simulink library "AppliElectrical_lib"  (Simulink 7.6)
settings: Solver=ode45  StartTime=0.0  StopTime=10.0  RelTol=1e-3
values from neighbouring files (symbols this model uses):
  A = [1+j -(1-j);1 -2/(1-j)]    [systeme_AX_B_phaseurs.m]
undefined symbols (not defined in the file or in its folder): AppliElectrical, erreur, F, gcbh, Giacolleto_NPN, model_FET_canal_N, nesl_callback, Ohm, PID_analogique, s, Transistor_NPN, V, vb2c, vb2e

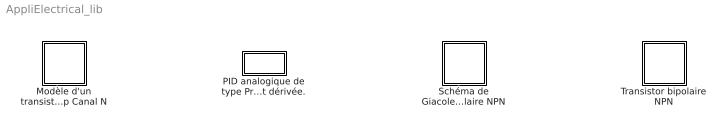
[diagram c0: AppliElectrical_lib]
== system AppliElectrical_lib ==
  Modèle d'un transistor à effet de champ Canal N : Subsystem  DialogController=NetworkEngine.DynNeDlgSource  LoadFcn=nesl_callback('LoadFcn',gcbh);  mask(Modèle d'un
transistor à effet
de champ Canal N){ComponentPath=AppliElectrical.model_FET_canal_N, ClassName=model_FET_canal_N, SchemaVersion=1, g=0.003, g_unit=A/V, rho=1e+6, rho_unit=Ohm, ie_Log=off, vgs_Log=off, is_Log=off, vds_Log=off, LocalVarNames=\, LocalVarDescs=ie\, LocalVarLogging=vgs\}
      mask help: Le modèle qui définit ce transistor spécifie: - la résistance Rgs entre la grille et la source, - la conductance g ou pente g=dId/dVgs, - sa résistance rho en parallèle à la source de courant g Vds.
      mask init:
      | nesl_preinitmask (gcb);
  "PID analogique de type Proportionnel, Intégral et dérivée." : Subsystem  DialogController=NetworkEngine.DynNeDlgSource  LoadFcn=nesl_callback('LoadFcn',gcbh);  mask(PID analogique de
type Proportionnel,
Intégral et dérivée.){ComponentPath=AppliElectrical.PID_analogique, ClassName=PID_analogique, SchemaVersion=1, Kp=10, Kp_unit=1, Ki=0.5, Ki_unit=1/s, Kd=0.01, Kd_unit=s, deriv_Log=off, erreur_Log=off, LocalVarNames=\, LocalVarDescs=deriv\, LocalVarLogging=erreur}
      mask prompts: Kp "Gain proportionnel"; Ki "Gain intégral"; Kd "Gain dérivée"
      mask help: L'entrée, err, de ce composant est l'erreur consigne-sortie. La sortie, cde, est la variation de commande. De fait, ce composant doit être suivi d'un intégrateur pour obtenir la commande à appliquer au processus
      mask init:
      | nesl_preinitmask (gcb);
  Schéma de Giacoletto d'un transistor bipolaire NPN : Subsystem  DialogController=NetworkEngine.DynNeDlgSource  LoadFcn=nesl_callback('LoadFcn',gcbh);  mask(Schéma de Giacoletto
d'un transistor
bipolaire NPN){ComponentPath=AppliElectrical.Giacolleto_NPN, ClassName=Giacolleto_NPN, SchemaVersion=1, Cbe=8e-11, Cbe_unit=F, Cbc=1e-11, Cbc_unit=F, h11=1000, h11_unit=Ohm, rbb=100, rbb_unit=Ohm, h21=100, h21_unit=1, g=1e-5, g_unit=1/Ohm, vb2e_Log=off, vb2c_Log=off, Ib_Log=off, Vbe_Log=off, Ic_Log=off, Vce_Log=off, LocalVarNames=\, LocalVarDescs=vb2e\, LocalVarLogging=vb2c\}
      mask prompts: Cbe "Capacitance Cb'e"; Cbc "Capacitance Cb'c"; h11 "résistance h11"; rbb "résistance rbb'"; h21 "gain en tension Ic=h21 Ib"; g "conductance 1/h22"
      mask help: Le schéma de Giacoletto modélise les transistors en hautes fréquences. Le modèle a besoin des paramètres suivants:
      mask init:
      | nesl_preinitmask (gcb);
  Transistor bipolaire NPN : Subsystem  DialogController=NetworkEngine.DynNeDlgSource  LoadFcn=nesl_callback('LoadFcn',gcbh);  mask(Transistor bipolaire
NPN){ComponentPath=AppliElectrical.Transistor_NPN, ClassName=Transistor_NPN, SchemaVersion=1, s=1e-6, s_unit=1/Ohm, h21=200, h21_unit=1, h12=1e-4, h12_unit=1, h11=1000, h11_unit=Ohm, Ib_Log=off, Vbe_Log=off, Ic_Log=off, Vce_Log=off, LocalVarNames=\, LocalVarDescs=Ib\, LocalVarLogging=Vbe\}
      mask prompts: s "1/h22"; h21 "Gain en courant h21"; h12 "Gain en tension inverse"; h11 "Résistance d'entrée h11"
      mask help: Le modèle qui définit ce transistor spécifie: - la résistance 1/h22 (s) entre le collecteur et l'émetteur - le gain en courant h21, - le paramètre h12, amplification inverse en tension - sa résistance d'entrée h11.
      mask init:
      | nesl_preinitmask (gcb);

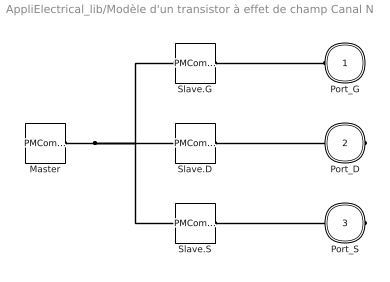
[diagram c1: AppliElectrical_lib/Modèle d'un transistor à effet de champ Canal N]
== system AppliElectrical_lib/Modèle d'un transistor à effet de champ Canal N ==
  Master : PMComponent  Tag=AppliElectrical.model_FET_canal_N  PhysicalDomain=network_engine_domain  SubClassName=master  LeftPortType=generic  RightPortType=generic  RConnTagsString=RConn1
  Slave.D : PMComponent  Tag=D  PhysicalDomain=network_engine_domain  SubClassName=terminal  LeftPortType=generic  RightPortType=foundation.electrical.electrical  LConnTagsString=LConn1  RConnTagsString=RConn1
  Slave.G : PMComponent  Tag=G  PhysicalDomain=network_engine_domain  SubClassName=terminal  LeftPortType=generic  RightPortType=foundation.electrical.electrical  LConnTagsString=LConn1  RConnTagsString=RConn1
  Slave.S : PMComponent  Tag=S  PhysicalDomain=network_engine_domain  SubClassName=terminal  LeftPortType=generic  RightPortType=foundation.electrical.electrical  LConnTagsString=LConn1  RConnTagsString=RConn1
  Port_G : PMIOPort  Tag=G  Port=1  Side=Left
  Port_D : PMIOPort  Tag=D  Port=2  Side=Right
  Port_S : PMIOPort  Tag=S  Port=3  Side=Right
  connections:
  Slave.G/RConn1 -- Port_G/RConn1
  Slave.G/LConn1 -- Slave.D/LConn1 -- Master/RConn1 -- Slave.S/LConn1
  Slave.D/RConn1 -- Port_D/RConn1
  Slave.S/RConn1 -- Port_S/RConn1

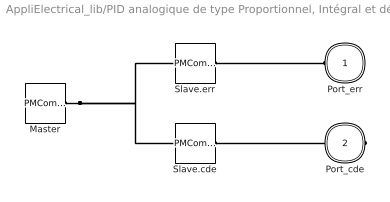
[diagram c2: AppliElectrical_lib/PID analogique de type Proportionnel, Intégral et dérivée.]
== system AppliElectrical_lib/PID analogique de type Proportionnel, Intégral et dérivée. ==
  Master : PMComponent  Tag=AppliElectrical.PID_analogique  PhysicalDomain=network_engine_domain  SubClassName=master  LeftPortType=generic  RightPortType=generic  RConnTagsString=RConn1
  Slave.cde : PMComponent  Tag=cde  PhysicalDomain=network_engine_domain  SubClassName=output  LeftPortType=generic  RightPortType=output  LConnTagsString=LConn1  RConnTagsString=RConn1
  Slave.err : PMComponent  Tag=err  PhysicalDomain=network_engine_domain  SubClassName=input  LeftPortType=generic  RightPortType=input  LConnTagsString=LConn1  RConnTagsString=RConn1
  Port_err : PMIOPort  Tag=err  Port=1  Side=Left
  Port_cde : PMIOPort  Tag=cde  Port=2  Side=Right
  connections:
  Slave.err/RConn1 -- Port_err/RConn1
  Master/RConn1 -- Slave.err/LConn1 -- Slave.cde/LConn1
  Slave.cde/RConn1 -- Port_cde/RConn1

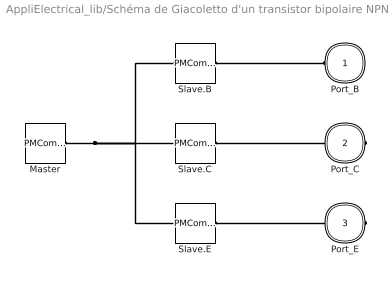
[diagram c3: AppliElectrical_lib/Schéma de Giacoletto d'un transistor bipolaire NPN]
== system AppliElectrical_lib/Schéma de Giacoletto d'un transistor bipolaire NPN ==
  Master : PMComponent  Tag=AppliElectrical.Giacolleto_NPN  PhysicalDomain=network_engine_domain  SubClassName=master  LeftPortType=generic  RightPortType=generic  RConnTagsString=RConn1
  Slave.B : PMComponent  Tag=B  PhysicalDomain=network_engine_domain  SubClassName=terminal  LeftPortType=generic  RightPortType=foundation.electrical.electrical  LConnTagsString=LConn1  RConnTagsString=RConn1
  Slave.C : PMComponent  Tag=C  PhysicalDomain=network_engine_domain  SubClassName=terminal  LeftPortType=generic  RightPortType=foundation.electrical.electrical  LConnTagsString=LConn1  RConnTagsString=RConn1
  Slave.E : PMComponent  Tag=E  PhysicalDomain=network_engine_domain  SubClassName=terminal  LeftPortType=generic  RightPortType=foundation.electrical.electrical  LConnTagsString=LConn1  RConnTagsString=RConn1
  Port_B : PMIOPort  Tag=B  Port=1  Side=Left
  Port_C : PMIOPort  Tag=C  Port=2  Side=Right
  Port_E : PMIOPort  Tag=E  Port=3  Side=Right
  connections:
  Slave.B/RConn1 -- Port_B/RConn1
  Slave.B/LConn1 -- Slave.C/LConn1 -- Master/RConn1 -- Slave.E/LConn1
  Slave.C/RConn1 -- Port_C/RConn1
  Slave.E/RConn1 -- Port_E/RConn1

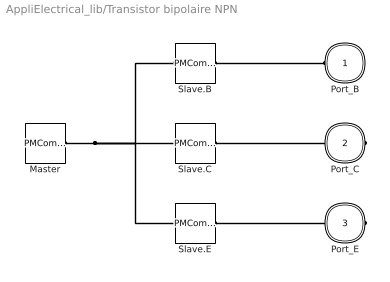
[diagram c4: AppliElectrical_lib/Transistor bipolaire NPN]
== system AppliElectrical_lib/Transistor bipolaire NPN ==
  Master : PMComponent  Tag=AppliElectrical.Transistor_NPN  PhysicalDomain=network_engine_domain  SubClassName=master  LeftPortType=generic  RightPortType=generic  RConnTagsString=RConn1
  Slave.B : PMComponent  Tag=B  PhysicalDomain=network_engine_domain  SubClassName=terminal  LeftPortType=generic  RightPortType=foundation.electrical.electrical  LConnTagsString=LConn1  RConnTagsString=RConn1
  Slave.C : PMComponent  Tag=C  PhysicalDomain=network_engine_domain  SubClassName=terminal  LeftPortType=generic  RightPortType=foundation.electrical.electrical  LConnTagsString=LConn1  RConnTagsString=RConn1
  Slave.E : PMComponent  Tag=E  PhysicalDomain=network_engine_domain  SubClassName=terminal  LeftPortType=generic  RightPortType=foundation.electrical.electrical  LConnTagsString=LConn1  RConnTagsString=RConn1
  Port_B : PMIOPort  Tag=B  Port=1  Side=Left
  Port_C : PMIOPort  Tag=C  Port=2  Side=Right
  Port_E : PMIOPort  Tag=E  Port=3  Side=Right
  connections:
  Slave.B/RConn1 -- Port_B/RConn1
  Slave.B/LConn1 -- Slave.C/LConn1 -- Master/RConn1 -- Slave.E/LConn1
  Slave.C/RConn1 -- Port_C/RConn1
  Slave.E/RConn1 -- Port_E/RConn1
